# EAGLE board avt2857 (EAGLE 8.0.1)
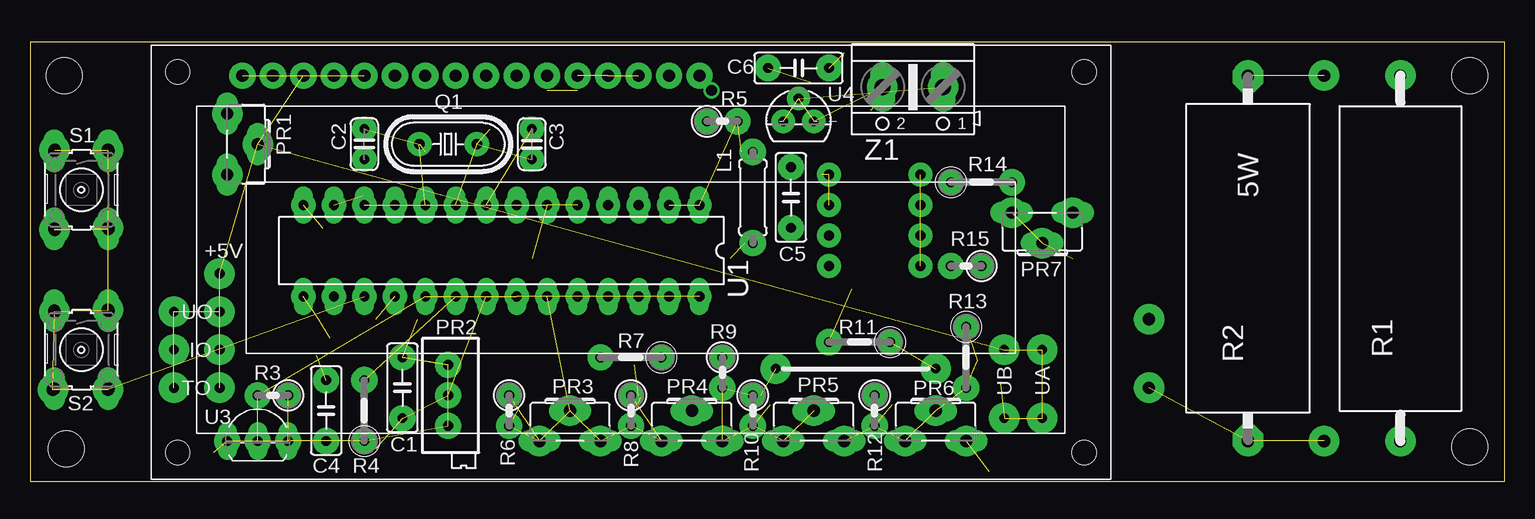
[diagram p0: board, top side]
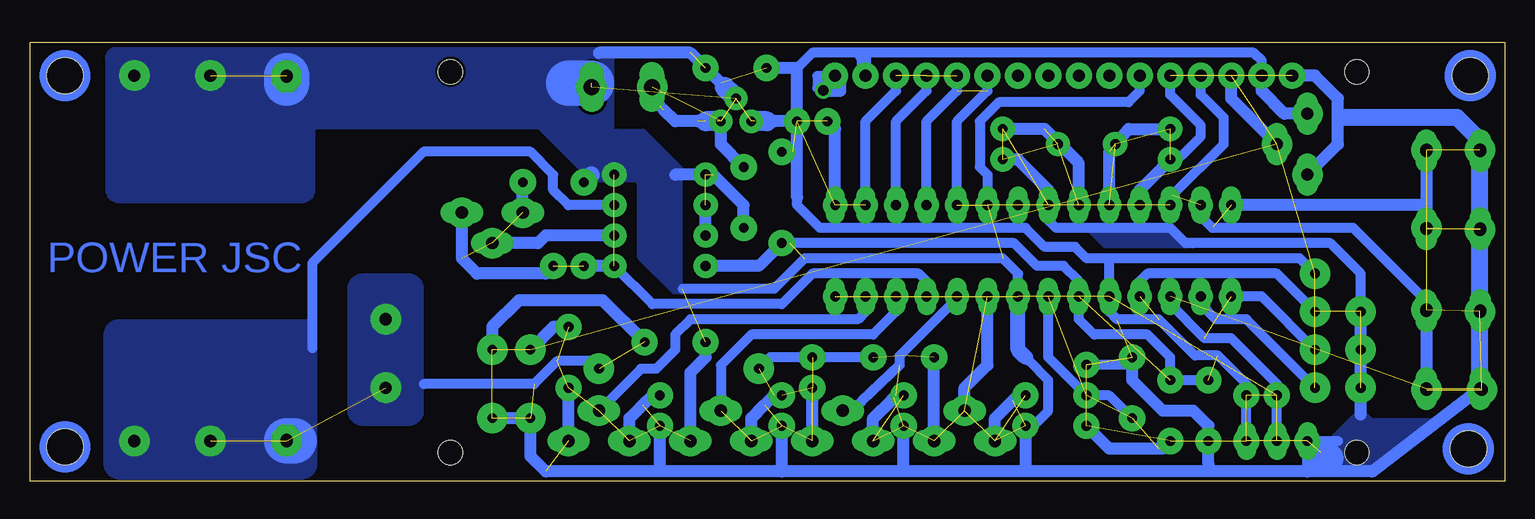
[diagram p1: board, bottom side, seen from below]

Size 122.92 x 36.61 mm. Coordinates in mm from the lower left corner, seen from the top.
Outline: 0,0 122.92,0 122.92,36.61 0,36.61 0,0
Copper layers (1*16): Top 0.035mm / dielectric 1.5mm / Bottom 0.035mm
Design rules "default": minimum track width 10mil, minimum drill 24mil, track to track 8mil, track to pad 8mil, pad to pad 8mil, via to via 8mil, smd to smd 8mil, copper to edge 1mil, drill to drill 8mil, minimum pad ring 15mil, minimum via ring 8mil, stop-mask expansion 4mil, vias tented up to drill 0mil, thermal gap 10mil
Holes 3 mm at 2.85,33.82 3.01,2.71 120.01,2.87 120.01,33.82

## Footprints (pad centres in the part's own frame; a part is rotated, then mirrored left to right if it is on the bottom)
C050-025X075 = drill 0.813 octagon: 1 -2.54,0; 2 2.54,0
C025-024X044 = drill 0.813 octagon: 1 -1.27,0; 2 1.27,0
LCD = drill 1.016 pad 1.676: 1 -33.02,15.875; 2 -30.48,15.875; 3 -27.94,15.875; 4 -25.4,15.875; 5 -22.86,15.875; 6 -20.32,15.875; 7 -17.78,15.875; 8 -15.24,15.875; 9 -12.7,15.875; 10 -10.16,15.875; 11 -7.62,15.875; 12 -5.08,15.875; 13 -2.54,15.875; 14 0,15.875; 15 2.54,15.875; 16 5.08,15.875 | hole 2: -38.417,16.192; -38.417,-15.557; 37.148,16.192; 37.148,-15.557
0207/7 = drill 0.813 octagon: 1 -3.81,0; 2 3.81,0
CA6H = drill 1.016 long: A -2.54,0; E 2.54,0; S 0,2.54
RTRIMT93XA = drill 0.61: 1 0,-2.54; 2 0,0; 3 0,2.54
HC49U-V = drill 0.813: 1 -2.413,0; 2 2.413,0
KH208-8 = drill 1.016 pad 2.54 octagon: 1 -13.875,0; 2 16.415,0
0207/2V = drill 0.813 octagon: 1 -1.27,0; 2 1.27,0
0207/5V = drill 0.813 octagon: 1 -2.54,0; 2 2.54,0
B3F-10XX = drill 1.016 long: 1 -3.251,2.261; 2 3.251,2.261; 3 -3.251,-2.261; 4 3.251,-2.261
DIL28-3 = drill 0.813 long: 1 -16.51,-3.81; 2 -13.97,-3.81; 3 -11.43,-3.81; 4 -8.89,-3.81; 5 -6.35,-3.81; 6 -3.81,-3.81; 7 -1.27,-3.81; 8 1.27,-3.81; 9 3.81,-3.81; 10 6.35,-3.81; 11 8.89,-3.81; 12 11.43,-3.81; 13 13.97,-3.81; 14 16.51,-3.81; 15 16.51,3.81; 16 13.97,3.81; 17 11.43,3.81; 18 8.89,3.81; 19 6.35,3.81; 20 3.81,3.81; 21 1.27,3.81; 22 -1.27,3.81; 23 -3.81,3.81; 24 -6.35,3.81; 25 -8.89,3.81; 26 -11.43,3.81; 27 -13.97,3.81; 28 -16.51,3.81
TO92-EBC = drill 0.813 long: DQ 0,-1.27; GND -2.54,-1.27; VDD 2.54,-1.27
TO92 = drill 0.813 octagon: 1 -1.27,0; 2 0,1.905; 3 1.27,0
AK500/2 = drill 1.321 long: 1 -2.515,0; 2 2.515,0

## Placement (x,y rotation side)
C1  [C050-025X075]  31.04,7.79 90 top
C2  [C025-024X044]  27.87,28.11 90 top
C3  [C025-024X044]  41.84,28.11 270 top
C4  [C050-025X075]  24.7,5.88 90 top
C5  [C050-025X075]  63.43,23.66 270 top
C6  [C050-025X075]  64.06,34.46 0 top
E$8  [LCD]  50.73,17.95 0 top
L1  [0207/7]  60.26,23.66 270 top
PR1  10k  [CA6H]  16.44,28.11 270 top
PR2  [RTRIMT93XA]  34.86,7.16 180 top
PR3  10k  [CA6H]  45.02,3.35 0 top
PR4  10k  [CA6H]  55.18,3.35 0 top
PR5  10k  [CA6H]  65.34,3.35 0 top
PR6  10k  [CA6H]  75.5,3.35 0 top
PR7  10k  [CA6H]  84.39,22.39 180 top
Q1  [HC49U-V]  34.86,28.11 0 top
R2  [KH208-8]  101.53,17.31 90 top
R3  [0207/2V]  20.25,7.16 180 top
R4  [0207/5V]  27.87,5.88 90 top
R5  [0207/2V]  57.72,30.01 0 top
R6  [0207/2V]  39.94,5.88 270 top
R7  [0207/5V]  50.1,10.33 180 top
R8  [0207/2V]  50.1,5.88 270 top
R9  [0207/2V]  57.72,9.06 270 top
R10  [0207/2V]  60.26,5.88 270 top
R11  [0207/5V]  69.14,11.6 180 top
R12  [0207/2V]  70.42,5.88 270 top
R13  [0207/5V]  78.03,10.33 270 top
R14  [0207/5V]  79.31,24.93 0 top
R15  [0207/2V]  78.03,17.95 180 top
S1  S  [B3F-10XX]  4.28,24.3 270 top
S2  S  [B3F-10XX]  4.28,10.96 270 top
U1  MEGA8  [DIL28-3]  39.3,19.22 180 top
U3  DS18B20  [TO92-EBC]  18.98,4.62 0 top
U4  78L05Z  [TO92]  64.06,30.01 0 top
Z1  [AK500/2]  73.59,32.87 180 top

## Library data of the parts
C1-C6 L1 PR2 R3-R15 = rcl
E$8 R2 S1 S2 U1 U3 = 00-my_lib
PR1 PR3-PR7 = pot
Q1 = crystal
U4 = linear
Z1 = con-ptr500

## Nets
N$10: U1.2
S$1: C3.2 Q1.2 U1.9
S$2: C2.2 Q1.1 U1.10
S$3: C3.1 U1.8
S$4: R5.2 U1.1
S$5: C1.1 PR2.2 U1.21
S$6: C1.2 PR2.1
S$7: R4.2 U1.20
S$8: S1.2 S1.4
S$9: S2.2 S2.4 U1.17
S$10: R3.2 U1.19 U3.DQ
S$11: R3.1 U3.VDD
S$13: PR3.A R6.1
S$14: PR4.A R8.1
S$15: PR3.S U1.23
S$16: PR2.3 R4.1
S$18: PR4.E R9.2
S$19: PR7.A
S$20: PR7.E
S$22: PR7.S
S$28: C5.2
S$29: E$8.1 E$8.5
S$30: E$8.3 PR1.S
S$32: U4.2 Z1.1
S$33: U4.3 Z1.2
S$88: E$8.13 R14.1

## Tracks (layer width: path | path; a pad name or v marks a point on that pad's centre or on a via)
+  (via drill 1.02 pad 2.54)  (1 unrouted)
  Bottom 0.813: 74.23,23.03 78.03,23.03 79.31,24.3 79.31,25.57 81.21,27.47 90.1,27.47 99.39,18.18 99.39,11.09
  Bottom 3.81: 101.53,3.35 100.89,3.35
  other vias: 107.88,3.35 114.23,3.35
  pour Bottom (no thermals): 100.26,0.17 arc-90 98.99,1.44 98.99,13.51 115.5,13.51 arc-90 116.77,12.24 116.77,1.44 arc-90 115.5,0.17
S$1  (2 unrouted)
S$2  (2 unrouted)
S$3  (1 unrouted)
S$4  (1 unrouted)
S$5  (2 unrouted)
S$6  (1 unrouted)
S$7  (1 unrouted)
S$8  (1 unrouted)
S$9  (2 unrouted)
S$10  (2 unrouted)
S$11  (1 unrouted)
S$12
  Bottom 0.813: 53.2,33.9 53.2,35.4 53.6,35.4 | 53.7,35.4 53.6,35.4 | 53.6,35.4 53.6,33.8
S$13  (1 unrouted)
S$14  (1 unrouted)
S$15  (1 unrouted)
S$16  (1 unrouted)
S$17  (via drill 0.81 pad 2.54)
  other vias: 16.44,25.57
S$18  (1 unrouted)
S$21
  Bottom 1.422: 13.58,30.33 3.96,30.33 2.06,28.43 2.06,21.12
S$23  (via drill 0.9)
  other vias: 56.8,32.6
S$24  (via drill 0.81 pad 1.93, 0.81 pad 2.18, 0.81 pad 2.54)  (7 unrouted)
  Bottom 1.016: 70.42,31.28 70.89,31.76 71.05,31.92 v71.05,32.87 | 70.1,30.97 69.14,30.01 67.24,30.01 | v65.34,30.01 65.34,28.11 v63.43,26.2
  Bottom 1.676: 65.65,30.01 66.61,30.01 | 61.53,30.01 62.48,30.01
  other vias: 64.06,31.92 62.8,30.01
S$25  (via drill 0.81 pad 2.03, 0.81 pad 2.18)  (4 unrouted)
  Bottom 0.813: 50.73,32.55 50.73,32.87 | 50.73,32.55 v50.73,33.82 | 50.73,32.55 53.27,30.01 v53.27,23.03
  Bottom 1.016: 59.3,27.47 v60.26,27.47 | v56.45,30.01 55.81,29.38 v55.81,23.03
  other vias: 48.19,33.82 58.98,30.01
S$26
  Bottom 0.813: 56.2,33.8 57.3,33.8 57.3,32.8 56.6,32.8 56.6,32.5 55.3,32.5 55.3,33.2
S$29  (1 unrouted)
S$30  (1 unrouted)
S$32  (1 unrouted)
S$33  (1 unrouted)
S$36  (via drill 0.81 pad 2.18)
  other vias: 17.71,33.82
S$37  (via drill 0.81 pad 2.18)
  other vias: 20.25,33.82
S$38  (via drill 0.81 pad 2.18)
  other vias: 22.79,33.82
S$39  (via drill 0.81 pad 2.18)
  other vias: 27.87,33.82
S$40  (via drill 0.81 pad 2.18)
  other vias: 25.33,33.82
S$41  (via drill 0.81 pad 2.18)
  other vias: 30.41,33.82
S$42  (via drill 0.81 pad 2.18)
  other vias: 32.95,33.82
S$43  (via drill 0.81 pad 2.18)
  other vias: 43.11,33.82
S$44  (via drill 0.81 pad 2.18)
  other vias: 45.65,33.82
S$47  (via drill 0.81 pad 2.18)
  other vias: 53.27,33.82
S$48  (via drill 0.81 pad 2.18)
  other vias: 55.81,33.82
S$49  (via drill 0.81 pad 2.18)
  other vias: 35.49,33.82
S$50  (via drill 0.81 pad 2.18)
  other vias: 40.57,33.82
S$51  (via drill 0.81 pad 2.18)
  other vias: 38.03,33.82
S$52  (via drill 0.81 pad 2.54)
  other vias: 16.44,30.65
S$53  (via drill 0.81 pad 2.54)  (11 unrouted)
  other vias: 18.98,28.11 15.8,7.79 15.8,10.96 11.99,10.96 11.99,7.79 84.39,5.25 81.21,5.25 84.39,10.96 81.21,10.96 11.99,14.14 15.8,14.14 15.8,17.31
S$57  (via drill 1.02 pad 2.54)  (7 unrouted)
  other vias: 6.5,27.63 2.06,27.63 2.06,20.97 6.5,21.12 6.5,14.3 6.5,7.63 1.9,7.63 2.06,14.14
S$58
  Bottom 0.813: 25.33,33.82 25.33,32.24 23.43,30.33 23.43,28.11 27.55,23.98
S$59
  Bottom 0.813: 27.87,33.82 27.87,32.24 25.33,29.7 25.33,28.74 26.92,27.16 27.55,27.16 28.19,26.52
S$62
  Bottom 1.016: 28.5,26.2 30.41,24.3 30.41,23.03
S$63
  Bottom 0.813: 30.41,33.82 30.41,32.55 31.36,31.6 42.16,31.6 43.75,30.01 43.75,26.2 43.11,25.57 43.11,23.98
S$68
  Bottom 0.813: 20.25,34.3 20.25,35.09 20.88,35.73 57.72,35.73 58.67,34.78
S$69
  Bottom 1.016: 61.53,34.46 58.98,34.46 58.98,29.06
S$70
  Bottom 1.016: 58.98,23.66 58.98,30.33
S$72
  Bottom 0.813: 58.98,23.35 58.98,23.03 57.08,21.12 39.94,21.12 38.35,19.54 35.81,19.54 34.86,18.58 17.07,18.58 15.8,17.31
S$73
  Bottom 0.813: 40.57,21.44 40.57,23.03
S$76
  Bottom 1.016: 6.5,23.03 22.79,23.03
S$77
  Bottom 1.016: 6.5,21.12 6.5,27.63
S$78
  Bottom 1.016: 30.41,21.44 30.41,23.03
S$81
  Bottom 1.016: 41.84,26.84 40.57,26.84 38.03,24.3 38.03,23.03
S$82
  Bottom 0.813: 32.95,15.41 32.95,18.27
S$83
  Bottom 0.813: 35.49,15.41 35.49,16.68 36.76,17.95 38.98,17.95 40.89,19.85 59.3,19.85
S$87
  Bottom 0.813: 48.19,15.41 48.19,16.68 48.83,17.31 57.72,17.31 60.26,14.78 71.05,14.78 74.23,17.95
S$88  (via drill 0.81 pad 2.03, 0.81 pad 2.18, 0.81 pad 2.54, 1.02 pad 2.54)  (81 unrouted)
  Bottom 0.813: 6.5,12.14 6.5,15 12.63,21.12 24.38,21.12 25.33,22.08 v25.33,23.03 | v50.73,23.03 50.73,30.01 48.19,32.55 E$8.13 | 27.71,23.82 27.87,23.66 v27.87,23.03 | v48.19,23.03 48.19,30.01 45.65,32.55 45.65,33.82 | 43.11,33.82 43.11,32.55 45.65,30.01 v45.65,23.03 | 68.51,16.04 60.89,16.04 58.35,18.58 41.84,18.58 40.57,17.31 v40.57,15.41 | v43.11,23.03 43.11,23.66 | v45.65,15.41 45.65,15.25 50.41,10.49 50.41,9.7 53.59,6.68 54.38,5.88 v55.18,5.88 | v75.5,9.38 76.13,10.01 78.99,10.01 80.89,8.11 90.1,8.11 | 13.9,3.35 v16.44,3.35 16.44,0.8 | v24.7,8.43 v27.87,8.43 | v32.95,15.41 32.95,14.14 32.31,13.51 28.82,13.51 25.81,10.49 23.9,10.49 21.52,8.11 v21.52,7.16 v21.52,3.35
  Bottom 1.016: v66.61,17.95 62.16,17.95 v60.26,19.85 59.62,19.85 | v39.94,7.16 40.57,7.16 41.05,6.68 | v70.42,7.16 71.05,7.16 71.84,6.36 | v50.1,7.16 50.73,7.16 50.89,7 | 28.82,2.71 28.5,2.71 v27.87,3.35 | v60.26,7.16 60.89,7.16 61.68,6.36 | 81.21,5.25 81.21,2.07 79.94,0.8 60.26,0.8 | 60.26,0.8 v60.26,4.62 | 60.26,0.8 16.44,0.8 11.04,0.8 2.22,7.63 | v66.61,20.49 v66.61,23.03 | 69.14,25.57 65.97,25.57 63.43,23.03 v63.43,21.12 | v81.84,22.39 v81.84,24.93 | v86.92,22.39 86.92,18.58 85.66,17.31 79.94,17.31 v79.31,17.95 | v74.23,17.95 v76.77,17.95 | 75.5,35.73 67.88,35.73 65.34,33.19 | 11.99,5.57 11.99,10.81 | v27.87,29.38 31.36,29.38 32.95,27.47 v32.95,23.03 | v41.84,29.38 38.35,29.38 35.49,26.52 v35.49,23.03
  Bottom 1.422: R14.1 76.13,25.57
  Bottom 2.54: 14.69,1.92 14.85,1.92 15.33,2.39
  Bottom 3.81: 76.13,33.19 78.03,33.19 | v101.53,33.82 101.53,33.19
  other vias: 22.79,23.03 27.87,26.84 30.41,23.03 41.84,26.84 66.61,11.6 38.03,23.03 40.57,23.03 30.41,15.41 35.49,15.41 55.81,15.41 39.94,4.62 53.27,15.41 38.03,15.41 50.73,15.41 42.48,3.35 45.02,5.88 48.19,15.41 43.11,15.41 47.55,3.35 52.64,3.35 50.1,4.62 47.55,10.33 52.64,10.33 65.34,5.88 67.88,3.35 70.42,4.62 34.86,4.62 34.86,7.16 72.95,3.35 71.69,11.6 75.5,5.88 34.86,9.7 31.04,5.25 31.04,10.33 78.03,12.87 78.03,7.79 57.72,10.33 57.72,7.79 18.98,7.16 62.16,9.38 24.7,3.35 78.03,3.35 57.72,3.35 62.8,3.35 18.98,3.35 66.61,25.57 84.39,19.85 74.23,25.57 74.23,23.03 74.23,20.49 66.61,34.46 61.53,34.46 76.77,24.93 93.28,7.79 93.28,13.51 76.13,32.87 107.88,33.82 114.23,33.82 101.53,3.35 37.24,28.11 32.47,28.11
  pour Bottom (no thermals): 91.37,17.31 95.18,17.31 arc-90 96.45,16.04 96.45,5.88 arc-90 95.18,4.62 91.37,4.62 arc-90 90.1,5.88 90.1,16.04 arc-90
  pour Bottom (isolate 0.254, no thermals): 68.51,24.93 68.51,15.63 69.37,15.63 69.37,15.64 72.14,18.41 arc45 72.32,18.84 72.32,24.93
  pour Bottom (isolate 0.254, no thermals): 68.51,24.3 68.51,26.2 71.69,29.38 74.23,29.38 74.23,36.21 115.98,36.21 arc-90 116.61,34.94 116.61,24.3 arc-90 115.5,23.19 100.26,23.19 arc-90 99.15,24.3 99.15,29.38 80.58,29.38 78.03,26.84
  pour Bottom (no thermals): 78.03,26.84 76.13,24.93 70.42,24.93 72.32,26.84
  pour Bottom (no thermals): 5.6,5.25 11.04,5.25 11.68,5.88 12.31,5.88 14.54,3.66 14.54,1.12 14.22,0.8 11.04,0.8
S$89
  Bottom 0.813: 30.41,15.41 30.41,16.68 29.77,17.31 18.98,17.31 15.8,14.14
S$90
  Bottom 0.813: 22.79,15.41 20.25,15.41 15.8,10.96
S$91  (via drill 0.81 pad 2.03)  (2 unrouted)
  Bottom 0.813: 15.8,7.79 21.52,13.51 24.06,13.51 25.33,14.78 v25.33,15.41 | 18.98,8.11 22.79,11.92 25.01,11.92 27.87,14.78 v27.87,15.41
  other vias: 22.79,15.41
S$94
  Bottom 0.813: 35.49,15.41 35.49,13.51 34.22,12.24 29.77,12.24 27.87,10.33 27.87,8.43
S$95
  Bottom 0.813: 31.04,5.25 32.95,7.16 34.86,7.16
S$96
  Bottom 0.813: 34.86,7.16 38.03,10.33 38.03,15.41
S$97
  Bottom 0.813: 39.62,10.01 38.03,8.43 38.03,5.88 39.3,4.62 39.94,4.62
  Bottom 1.016: 39.94,4.62 39.94,1.44
S$98
  Bottom 0.813: 62.16,9.38 61.21,10.33 57.72,10.33
S$99
  Bottom 0.813: 52.64,10.33 57.72,10.33
S$101
  Bottom 1.016: 20.25,33.98 20.25,32.55 18.34,30.65 16.44,30.65
S$102
  Bottom 1.016: 22.79,33.82 22.79,31.92 18.98,28.11
S$103
  Bottom 1.016: 17.71,33.82 15.8,33.82 13.9,31.92 13.9,28.11 16.44,25.57
S$104
  Bottom 1.016: 6.5,7.63 6.5,14.3
S$105
  Bottom 1.016: 11.99,10.96 11.99,14.14
S$107
  Bottom 1.016: 28.98,2.71 32.95,2.71 34.86,4.62
S$108
  Bottom 1.016: 24.7,3.03 24.7,4.62 25.96,5.88 28.5,5.88 31.04,8.43 31.04,10.33
S$109
  Bottom 1.016: 42.48,3.5 42.48,5.25 41.21,6.52
S$111
  Bottom 1.016: 81.21,5.25 84.39,5.25
S$112
  Bottom 1.016: 78.03,3.35 78.03,7.79
S$113
  Bottom 1.016: 72,6.2 72.95,5.25 72.95,3.35
S$114
  Bottom 1.016: 70.42,1.44 70.42,4.62
S$115
  Bottom 1.016: 66.61,11.6 66.61,10.33 67.88,9.06 67.88,3.35
S$116
  Bottom 1.016: 57.72,3.35 57.72,7.79
S$117
  Bottom 1.016: 61.68,6.36 62.8,5.25 62.8,3.35
S$118
  Bottom 1.016: 47.55,3.35 47.55,10.33
S$119
  Bottom 1.016: 51.05,6.84 52.64,5.25 52.64,3.35
S$120
  Bottom 1.016: 43.11,15.41 43.11,9.7 45.02,7.79 45.02,5.88
S$121
  Bottom 1.27: 40.57,15.25 40.57,10.96 39.94,10.33
S$122
  Bottom 1.016: 50.1,1.12 50.1,4.62
S$124
  Bottom 1.016: 24.7,1.44 24.7,3.03
S$125
  Bottom 0.813: 18.98,3.35 18.98,8.11
S$127
  Bottom 0.813: 31.2,9.7 34.86,9.7
S$128
  Bottom 0.813: 50.73,15.41 50.73,14.14 52.64,12.24 62.8,12.24 65.34,9.7 65.34,5.88
S$129
  Bottom 0.813: 53.27,15.41 53.27,14.14 53.91,13.51 67.88,13.51 69.14,12.24 69.14,10.96 70.73,9.38 72,9.38 75.5,5.88
S$130
  Bottom 1.016: 71.69,11.6 75.18,15.09 82.16,15.09 84.39,12.87 84.39,10.96
S$132
  Bottom 1.016: 84.23,19.85 80.58,19.85 79.94,20.49 74.23,20.49
S$133
  Bottom 1.016: 81.21,10.96 79.31,12.87 78.03,12.87
S$135
  Bottom 1.676: 64.38,32.24 65.02,32.87
S$138
  Bottom 1.016: 58.98,30.01 60.89,30.01
S$143
  Bottom 1.422: 2.06,13.51 2.06,20.81
S$144
  Bottom 0.813: 38.03,23.19 38.03,21.76 37.4,21.12 27.87,21.12 26.6,19.85 25.96,19.85 | 11.99,14.14 11.99,17.31 14.54,19.85 25.96,19.85 | 25.96,19.85 26.28,19.85
  pour Bottom (no thermals): 26.6,19.85 26.6,19.45 28.94,19.45 33.42,19.45 33.42,19.46 34.82,20.86 28.03,20.86 26.63,19.46
S$145
  Bottom 1.422: 2.06,7.79 2.06,12.87
(copper drawn outside any net)
  shapes: Bottom circle x4

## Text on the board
Bottom: POWER JSC
tNames: +5V | UO | IO | R1 | TO | UB | UA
